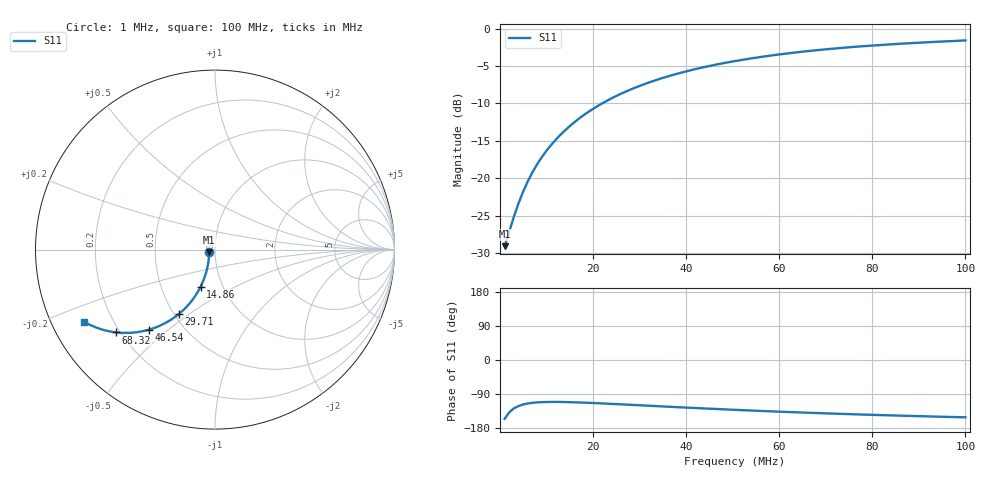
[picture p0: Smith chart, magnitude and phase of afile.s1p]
# Hz S RI R 50.0
! written by SimSmith version 18.3b
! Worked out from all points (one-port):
!   101 points, 1 MHz to 100 MHz, reference 50 ohm
!   lowest |S11| = -29.1 dB at 1 MHz (marker M1), VSWR 1.07, Z = 46.9 - j1.38 ohm
!   |S11| at or under -10 dB: start of sweep to 21.94 MHz
!   S11 on the Smith chart (normalised r, x): 1 MHz: 0.94, -0.03; 14.86 MHz: 0.79, -0.34; 29.71 MHz: 0.53, -0.46; 46.54 MHz: 0.32, -0.43; 68.32 MHz: 0.18, -0.35; 100 MHz: 0.10, -0.25
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1000000  -0.032 -0.0147
1990000  -0.0326 -0.0293
2980000  -0.0338 -0.0437
3970000  -0.0355 -0.0577
4960000  -0.0373 -0.0721
5950000  -0.0398 -0.0861
6940000  -0.0427 -0.1003
7930000  -0.0459 -0.1143
9910000  -0.054 -0.1417
1.189e7  -0.0629 -0.168
1.387e7  -0.0738 -0.1936
1.486e7  -0.0802 -0.2063
1.783e7  -0.1002 -0.2422
2.08e7  -0.1226 -0.2756
2.377e7  -0.1473 -0.306
2.575e7  -0.164 -0.325
2.971e7  -0.2005 -0.3581
3.466e7  -0.249 -0.393
3.862e7  -0.288 -0.4147
4.654e7  -0.3655 -0.4457
5.05e7  -0.4026 -0.4544
5.446e7  -0.4383 -0.4609
6.337e7  -0.5139 -0.464
6.832e7  -0.5515 -0.4613
7.525e7  -0.5996 -0.453
8.119e7  -0.6364 -0.4426
8.812e7  -0.6745 -0.4288
1e8  -0.7311 -0.4009
